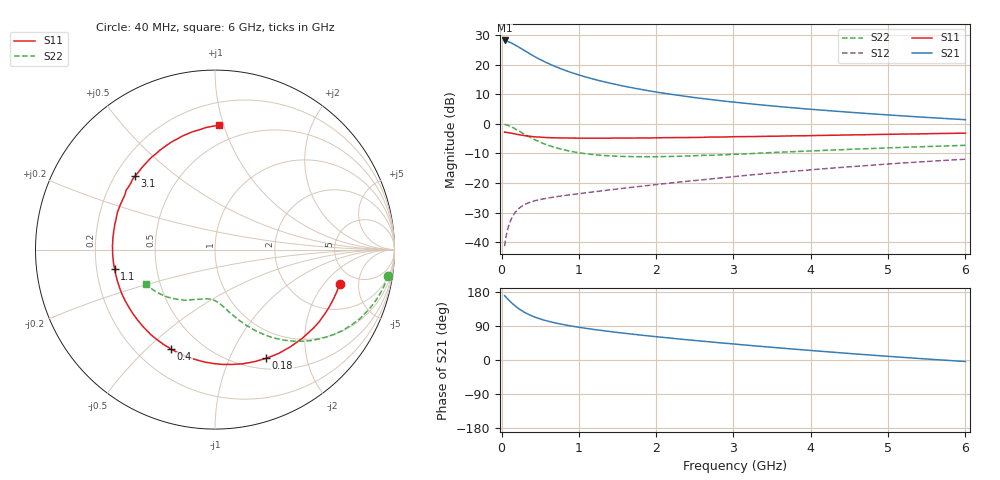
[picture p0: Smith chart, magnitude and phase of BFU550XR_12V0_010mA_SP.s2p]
! Filename:  P:\Prog\Test\Noise\ATS_data\Testdata_Net\03 Spar\BFU550XR_APG2013_45_C05_12p0V_010mA_SP_CM01_D.s2p
! Date/Time: Tue 06/Aug/2013 14:38:19
! BFU550XR_APG2013_45_C05_12p0V_1to35mA_SP_CM01_Bias5_R.s2p
! MDIF S-parameter v. bias file
! BFU550XR_APG2013_45_C05_12p0V_1to35mA_SP_CM01
! Date/time Fri Aug 02 14:58:10 2013
! VAR V_out= 12.0010
! VAR I_out= 10.0000
! VAR V_in= 0.7974
! VAR I_in= 0.0930
! Device data file deembeded for feedlines and parallel
! Original file: \03 Spar\BFU550XR_APG2013_45_C05_12p0V_010mA_SP_CM01_R.s2p
! Feed-files: PR006V01_02082013_Feed1.s2p, PR006V01_02082013_Feed2.s2p
! Parallel-file: PR006V01_02082013_Par.s2p
# MHz S MA R 50
!  Freq-MHz  S11-mag  S11-arg  S21-mag  S21-arg  S12-mag  S12-arg  S22-mag  S22-arg
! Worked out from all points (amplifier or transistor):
!   98 points, 40 MHz to 6 GHz, reference 50 ohm
!   highest |S21| = 28.1 dB at 40 MHz (marker M1)
!   |S21| within 3 dB of that: start of sweep to 270.5 MHz
!   unconditionally stable (mu >= 1): 2.004 GHz to 3.984 GHz
!   at 300 MHz: K = 0.28, MSG = 26.0 dB, |S12| = -27.3 dB
!   at 1.6 GHz: K = 0.93, MSG = 17.2 dB, |S12| = -21.7 dB
!   at 6 GHz: K = 0.87, MSG = 6.7 dB, |S12| = -12.0 dB
!   S11 on the Smith chart (normalised r, x): 40 MHz: 3.66, -2.96; 180 MHz: 0.63, -1.38; 400 MHz: 0.34, -0.60; 1.1 GHz: 0.28, -0.09; 3.1 GHz: 0.28, +0.36; 6 GHz: 0.36, +0.96
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40  0.7207 -15.7  25.51 170.0  0.008534 79.1  0.9723 -8.6
50  0.7178 -19.5  25.39 167.2  0.01063 78.2  0.9684 -10.9
80  0.7084 -30.9  24.52 161.1  0.01645 73.8  0.9402 -17.4
120  0.6934 -45.5  23.41 152.9  0.0235 67.8  0.8957 -25.3
140  0.6853 -52.2  22.71 149.1  0.02658 65.1  0.868 -29.0
180  0.6694 -64.9  21.23 142.1  0.03209 60.1  0.814 -35.5
220  0.6548 -76.3  19.85 135.9  0.03649 56.1  0.7598 -41.1
280  0.6347 -90.9  17.75 127.9  0.04169 51.2  0.6838 -48.4
340  0.6188 -103.4  15.92 121.3  0.04558 47.6  0.6176 -54.0
400  0.6057 -113.7  14.32 115.8  0.04857 45.0  0.5617 -58.8
500  0.5932 -127.2  12.15 108.5  0.05256 42.3  0.4891 -64.8
550  0.5871 -133.1  11.29 105.2  0.05393 41.4  0.4579 -67.4
650  0.5801 -142.3  9.816 100.0  0.05697 40.5  0.4131 -71.4
850  0.5735 -156.5  7.748 91.6  0.06202 40.2  0.3517 -77.7
1050  0.5706 -166.9  6.377 84.9  0.06693 41.2  0.3163 -82.5
1100  0.5695 -169.1  6.103 83.4  0.06821 41.5  0.3101 -83.6
1500  0.5715 176.1  4.545 72.7  0.07899 43.6  0.2825 -91.0
2050  0.5787 160.9  3.353 60.5  0.09511 45.7  0.2783 -99.8
3100  0.6052 137.6  2.251 40.5  0.1316 46.2  0.3072 -114.6
4100  0.6333 119.0  1.714 23.5  0.1706 42.7  0.351 -128.3
5200  0.6689 100.5  1.354 6.8  0.2174 36.2  0.3988 -143.0
6000  0.6934 88.3  1.17 -4.0  0.2511 30.2  0.4313 -153.7
